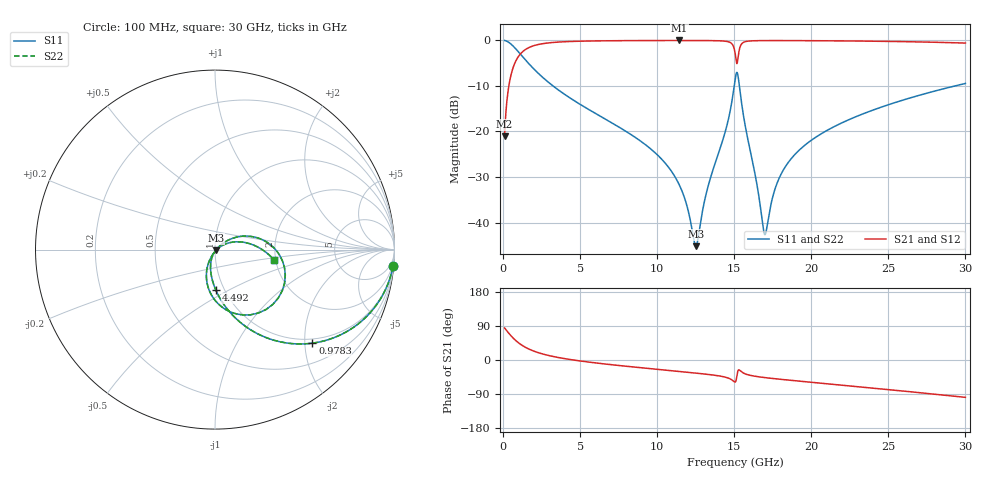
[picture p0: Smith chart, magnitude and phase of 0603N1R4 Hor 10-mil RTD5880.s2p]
# GHz S MA R 50
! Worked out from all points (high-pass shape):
!   3201 points, 100 MHz to 30 GHz, reference 50 ohm
!   highest |S21| = -0.05 dB at 11.44 GHz (marker M1); lowest = -21.0 dB at 100 MHz (marker M2)
!   |S21| within 3 dB of the highest: 1.113 GHz to 15.07 GHz (13.95 GHz wide, 172 % of centre); 15.28 GHz to end of sweep
!   lowest |S11| = -45.2 dB at 12.51 GHz (marker M3), VSWR 1.01, Z = 50.4 - j0.337 ohm
!   |S11| at or under -10 dB: 3.235 GHz to 15 GHz (11.76 GHz wide, 129 % of centre); 15.33 GHz to 29.34 GHz (14.01 GHz wide, 62.7 % of centre)
!   |S22| runs from -45.2 to 0.0 dB; largest |S21 - S12| = 0
!   S11 on the Smith chart (normalised r, x): 100 MHz: 1, -21; 978.3 MHz: 0.90, -2.17; 4.492 GHz: 0.91, -0.43; 30 GHz: 1.97, -0.26
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0.1  0.9958 -5.4  0.08878 84.5  0.08878 84.5  0.9958 -5.4
0.4550625  0.9264 -23.3  0.3752 66.6  0.3752 66.6  0.9264 -23.3
0.9783125  0.7528 -43.8  0.6571 46.1  0.6571 46.1  0.7528 -43.8
2.239719  0.4415 -69.9  0.8956 19.9  0.8956 19.9  0.4415 -69.9
4.491562  0.2244 -89.0  0.972 0.4  0.972 0.4  0.2244 -89.0
5.089563  0.1941 -92.2  0.9783 -3.0  0.9783 -3.0  0.1941 -92.2
10.06978  0.05418 -110.5  0.9943 -24.8  0.9943 -24.8  0.05418 -110.5
11.44331  0.02576 -109.7  0.9948 -30.2  0.9948 -30.2  0.02576 -109.7
12.5085  0.005512 -37.3  0.9943 -34.5  0.9943 -34.5  0.005512 -37.3
13.28403  0.02432 35.9  0.9928 -38.0  0.9928 -38.0  0.02432 35.9
14.39594  0.09647 34.9  0.9784 -45.0  0.9784 -45.0  0.09647 34.9
14.85378  0.2163 19.7  0.913 -52.7  0.913 -52.7  0.2163 19.7
15.05  0.3652 -5.8  0.734 -58.1  0.734 -58.1  0.3652 -5.8
15.27425  0.3785 -71.4  0.6958 -26.4  0.6958 -26.4  0.3785 -71.4
15.51719  0.1838 -104.4  0.9272 -32.5  0.9272 -32.5  0.1838 -104.4
15.97503  0.06897 -116.8  0.9819 -39.9  0.9819 -39.9  0.06897 -116.8
16.98416  0.007383 -45.5  0.9924 -46.4  0.9924 -46.4  0.007383 -45.5
17.58216  0.02155 22.9  0.9929 -49.1  0.9929 -49.1  0.02155 22.9
18.06803  0.03473 28.2  0.9928 -51.2  0.9928 -51.2  0.03473 28.2
20.03956  0.08084 26.5  0.99 -58.9  0.99 -58.9  0.08084 26.5
25.01978  0.1968 9.6  0.9725 -78.2  0.9725 -78.2  0.1968 9.6
30  0.3361 -10.1  0.9322 -98.6  0.9322 -98.6  0.3361 -10.1
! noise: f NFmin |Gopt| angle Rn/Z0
0.1  0.002586  0.9905  0.3097  0.06213
3.417  0.004079  0.8119  9.952  0.00449
6.743  0.006822  0.7826  19.03  0.006265
10.06  0.00951  0.7705  28.01  0.00796
13.39  0.01422  0.795  36.85  0.01292
16.7  0.01703  0.7894  45.7  0.01418
20.03  0.01654  0.7489  54.1  0.01058
23.35  0.01888  0.7473  62.31  0.01109
26.67  0.02157  0.7502  70.31  0.01175
30  0.02452  0.7555  78.1  0.01238
